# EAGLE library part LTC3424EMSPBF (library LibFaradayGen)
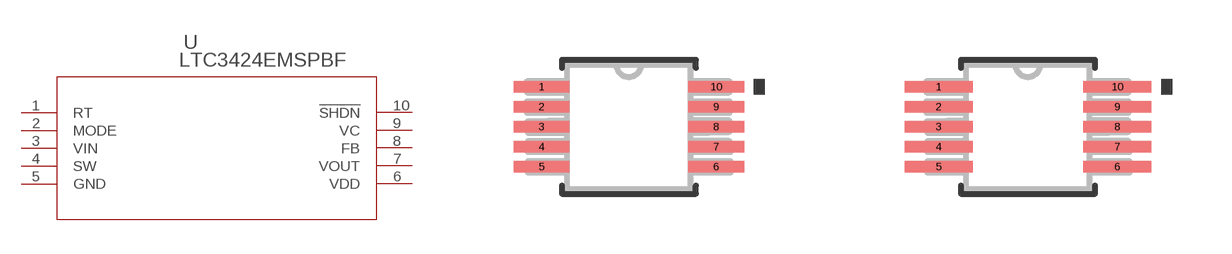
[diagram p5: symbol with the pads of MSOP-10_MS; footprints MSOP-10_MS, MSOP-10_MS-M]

Designator prefix U

## LTC3424EMSPBF (MANUFACTURER_PART_NUMBER: LTC3424EMS#PBF; VENDOR: Linear Technology)  [MSOP-10_MS]
1  RT  pas
2  MODE  pas
3  VIN  in
4  SW  pas
5  GND  pwr
6  VDD  pwr
7  VOUT  out
8  FB  out
9  VC  out
10  !SHDN  out

## LTC3424EMSPBFMSOP-10_MS-M (MANUFACTURER_PART_NUMBER: LTC3424EMS#PBF; VENDOR: Linear Technology)  [MSOP-10_MS-M]
Pads as for MSOP-10_MS

## LTC3424EMSPBFMSOP-10_MS-L (MANUFACTURER_PART_NUMBER: LTC3424EMS#PBF; VENDOR: Linear Technology)  [MSOP-10_MS-L]
Pads as for MSOP-10_MS

## Footprint MSOP-10_MS (pad centres in mm)
smd 1.397 x 0.279: 1 -2.184,1.001; 2 -2.184,0.5; 3 -2.184,0; 4 -2.184,-0.5; 5 -2.184,-1.001; 6 2.184,-1.001; 7 2.184,-0.5; 8 2.184,0; 9 2.184,0.5; 10 2.184,1.001

## Footprint MSOP-10_MS-M (pad centres in mm)
smd 1.702 x 0.279: 1 -2.235,1.001; 2 -2.235,0.5; 3 -2.235,0; 4 -2.235,-0.5; 5 -2.235,-1.001; 6 2.235,-1.001; 7 2.235,-0.5; 8 2.235,0; 9 2.235,0.5; 10 2.235,1.001

## Footprint MSOP-10_MS-L (pad centres in mm)
smd 1.092 x 0.279: 1 -2.134,1.001; 2 -2.134,0.5; 3 -2.134,0; 4 -2.134,-0.5; 5 -2.134,-1.001; 6 2.134,-1.001; 7 2.134,-0.5; 8 2.134,0; 9 2.134,0.5; 10 2.134,1.001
